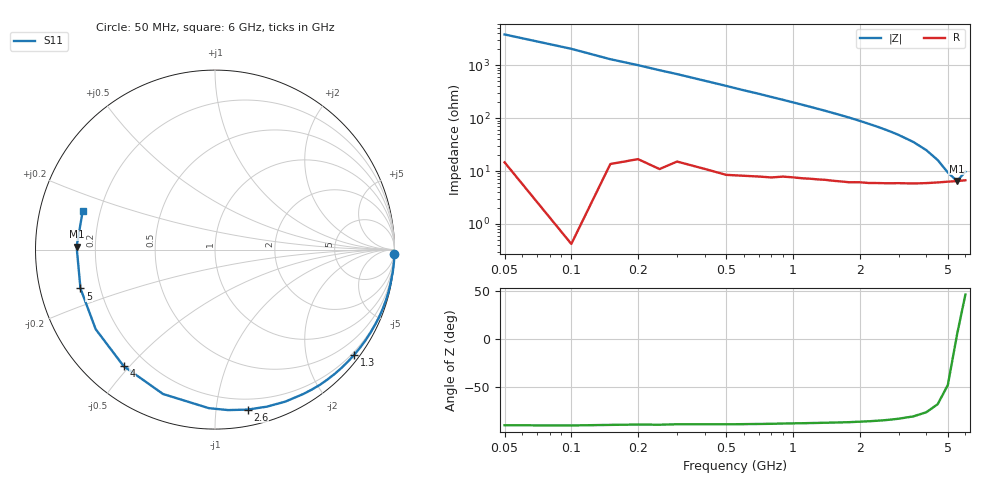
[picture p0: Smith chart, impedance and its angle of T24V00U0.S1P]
! SIEMENS Discrete & RF Semiconductors
! BAS70-04W
! Si Schottky Diode in SOT323
! VR = 4 V
! S-Parameters:  November  1997
# GHz  S  MA  R  50
!  f  S11
! GHz  MAG  ANG
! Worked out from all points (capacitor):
!   34 points, 50 MHz to 6 GHz, reference 50 ohm
!   read as one part to ground: C = 815 fF near 50 MHz
!   lowest |Z| = 6.48 ohm at 5.5 GHz (marker M1)
!   series resonance near 5.466 GHz, so ESL is about 1 nH
!   S11 on the Smith chart (normalised r, x): 50 MHz: 0, -76; 1.3 GHz: 0.14, -2.98; 2.6 GHz: 0.12, -1.22; 4 GHz: 0.12, -0.48; 5 GHz: 0.13, -0.14; 6 GHz: 0.13, +0.14
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0.05  0.9999 -1.5
0.1  1 -2.8
0.15  0.9992 -4.4
0.25  0.9983 -7.1
0.5  0.995 -14.0
0.6  0.993 -16.9
0.7  0.9909 -19.6
0.8  0.9885 -22.5
0.9  0.985 -25.3
1.1  0.9792 -31.1
1.2  0.9758 -34.0
1.3  0.9724 -37.0
1.4  0.9687 -39.9
1.5  0.9652 -43.0
1.6  0.9615 -46.0
1.8  0.9535 -52.2
2  0.9428 -58.6
2.2  0.9331 -65.2
2.4  0.9216 -71.7
2.6  0.9097 -78.5
2.8  0.8972 -85.3
3  0.8841 -92.2
3.5  0.8551 -109.8
4  0.825 -128.1
4.5  0.7991 -146.3
5  0.7801 -163.9
5.5  0.7712 178.8
6  0.7678 163.7
